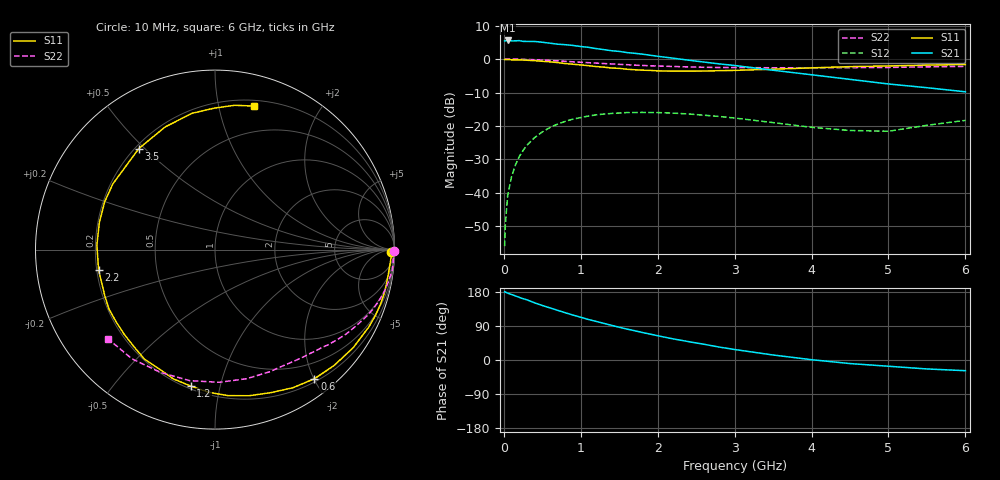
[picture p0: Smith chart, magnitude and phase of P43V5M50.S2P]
! SIEMENS Small Signal Semiconductors
! BFP182
! Si NPN RF Bipolar Junction Transistor in SOT143
! VCE = 3.5 V  IC = 0.5 mA
! Common Emitter S-Parameters:  March  1996
# GHz  S  MA  R  50
!  f  S11  S21  S12  S22
! GHz  MAG  ANG  MAG  ANG  MAG  ANG  MAG  ANG
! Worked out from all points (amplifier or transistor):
!   36 points, 10 MHz to 6 GHz, reference 50 ohm
!   highest |S21| = 5.6 dB at 50 MHz (marker M1)
!   |S21| within 3 dB of that: start of sweep to 1.379 GHz
!   unconditionally stable (mu >= 1): 2.959 GHz to end of sweep
!   at 250 MHz: K = 0.08, MSG = 16.3 dB, |S12| = -27.3 dB
!   at 1.4 GHz: K = 0.49, MSG = 9.4 dB, |S12| = -16.3 dB
!   at 6 GHz: K = 1.22, MAG = 1.4 dB, |S12| = -18.3 dB
!   S11 on the Smith chart (normalised r, x): 10 MHz: 70, -56; 600 MHz: 0.24, -2.01; 1.2 GHz: 0.22, -0.81; 2.2 GHz: 0.21, -0.08; 3.5 GHz: 0.21, +0.48; 6 GHz: 0.25, +1.27
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0.01  0.9826 -0.8  1.865 179.7  0.0016 93.8  0.9999 -0.3
0.02  0.9842 -1.5  1.874 179.3  0.0034 94.6  0.992 -0.6
0.05  0.9788 -4.5  1.895 176.4  0.0092 88.1  0.998 -1.6
0.1  0.975 -8.8  1.868 172.9  0.0174 84.4  0.9946 -3.2
0.2  0.9714 -17.9  1.883 165.4  0.0348 78.7  0.9946 -6.4
0.3  0.9596 -26.6  1.834 158.8  0.0515 72.5  0.9853 -9.5
0.4  0.9444 -35.3  1.83 150.9  0.0671 67.1  0.9769 -12.5
0.6  0.9081 -52.4  1.725 137.5  0.095 56.0  0.9521 -18.3
0.8  0.8558 -68.6  1.638 124.6  0.1172 46.1  0.9247 -23.4
0.9  0.836 -76.9  1.596 118.5  0.1268 41.3  0.9087 -25.9
1.1  0.7953 -92.7  1.497 106.9  0.1408 32.7  0.8816 -30.4
1.2  0.7721 -100.1  1.433 101.9  0.1465 28.4  0.8696 -32.7
1.6  0.7042 -130.0  1.248 81.6  0.1588 14.7  0.8239 -40.1
1.9  0.677 -150.8  1.141 68.4  0.1587 6.0  0.7937 -45.5
2.2  0.6586 -170.1  1.03 55.8  0.1555 -1.3  0.7742 -50.6
2.8  0.67 156.5  0.846 34.1  0.1387 -12.4  0.7475 -61.6
3.5  0.7051 127.0  0.68 13.2  0.1123 -18.3  0.7406 -76.2
4  0.7378 112.1  0.582 0.8  0.0954 -15.2  0.7396 -88.1
4.5  0.7701 99.5  0.497 -9.4  0.0856 -7.3  0.7437 -100.9
5  0.7885 90.2  0.424 -16.5  0.0834 7.5  0.7487 -113.9
5.5  0.8116 82.2  0.373 -23.6  0.1024 14.3  0.7646 -127.3
6  0.8283 74.9  0.324 -28.2  0.1212 15.7  0.7762 -140.3
